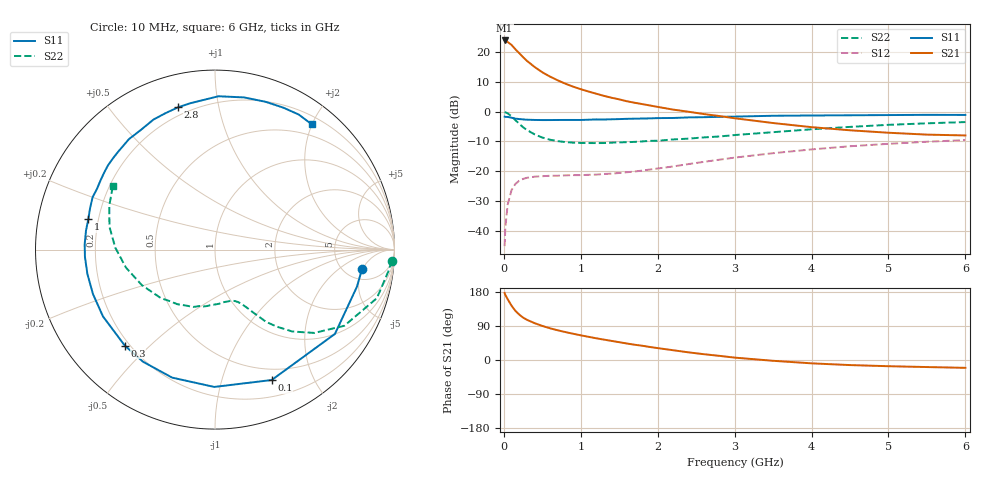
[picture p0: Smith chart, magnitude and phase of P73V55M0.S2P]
! SIEMENS Small Signal Semiconductors
! BFP196
! Si NPN RF Bipolar Junction Transistor in SOT143
! VCE = 3.5 V  IC = 5 mA
! Common Emitter S-Parameters:  May  1996
# GHz  S  MA  R  50
!  f  S11  S21  S12  S22
! GHz  MAG  ANG  MAG  ANG  MAG  ANG  MAG  ANG
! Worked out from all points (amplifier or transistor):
!   36 points, 10 MHz to 6 GHz, reference 50 ohm
!   highest |S21| = 23.9 dB at 10 MHz (marker M1)
!   |S21| within 3 dB of that: start of sweep to 151.6 MHz
!   unconditionally stable (mu >= 1): 1.13 GHz to 3.175 GHz
!   at 250 MHz: K = 0.25, MSG = 20.5 dB, |S12| = -22.6 dB
!   at 1.4 GHz: K = 1.15, MAG = 10.4 dB, |S12| = -20.8 dB
!   at 6 GHz: K = 1.00, MSG = 0.8 dB, |S12| = -9.5 dB
!   S11 on the Smith chart (normalised r, x): 10 MHz: 7.16, -4.86; 100 MHz: 0.37, -1.46; 300 MHz: 0.18, -0.42; 1 GHz: 0.16, +0.12; 2.8 GHz: 0.16, +0.76; 6 GHz: 0.32, +1.99
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0.01  0.8262 -7.5  15.75 176.9  0.0055 88.3  0.9862 -3.6
0.02  0.8176 -14.6  15.3 171.6  0.0116 84.0  0.9748 -6.9
0.05  0.8168 -35.1  14.84 160.3  0.0275 72.0  0.9416 -16.7
0.1  0.7923 -66.5  13.25 143.4  0.0481 58.1  0.8362 -30.5
0.15  0.7652 -90.3  11.2 129.7  0.0611 46.6  0.7222 -40.0
0.2  0.7522 -108.5  9.651 119.9  0.0692 39.0  0.6268 -46.7
0.25  0.7424 -122.7  8.245 111.9  0.0742 33.4  0.548 -51.4
0.3  0.734 -133.2  7.158 106.1  0.0775 30.2  0.4932 -54.7
0.4  0.7267 -149.2  5.643 97.2  0.081 25.3  0.4158 -58.4
0.5  0.7236 -160.0  4.595 89.9  0.0825 22.8  0.3679 -61.3
0.6  0.7238 -169.2  3.892 83.7  0.0838 22.0  0.3381 -63.8
0.7  0.7258 -176.8  3.368 78.4  0.084 21.3  0.3203 -66.1
0.8  0.7267 177.6  2.955 73.7  0.0851 21.4  0.3086 -68.5
1  0.7261 166.3  2.389 65.1  0.0859 23.0  0.2984 -73.4
1.1  0.7335 161.5  2.184 61.2  0.087 24.3  0.2973 -76.4
1.6  0.759 141.8  1.498 43.5  0.0961 32.0  0.3076 -91.9
2.2  0.7842 121.8  1.085 25.8  0.1202 39.1  0.3418 -110.8
2.8  0.819 104.5  0.846 11.0  0.156 39.7  0.3832 -131.7
3.5  0.8546 88.7  0.645 -2.1  0.2008 34.6  0.4528 -154.0
4.5  0.8705 71.0  0.487 -13.4  0.2627 23.2  0.5556 178.9
5.5  0.8854 58.2  0.412 -18.6  0.3128 10.6  0.6379 157.4
6  0.882 52.4  0.399 -20.7  0.3335 3.9  0.6697 148.2
